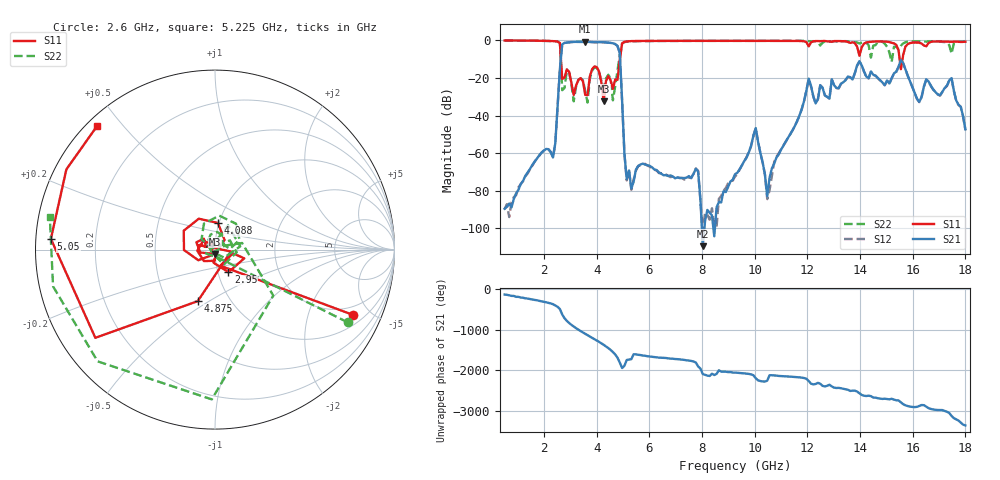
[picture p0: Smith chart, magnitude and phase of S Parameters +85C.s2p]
!Agilent Technologies,N5230A,MY45001468,A.07.50.67
!Agilent N5230A: A.07.50.67
!Date: Thursday, June 27, 2024 16:47:59
!Correction: S11(Full 2 Port(1,2))
!S21(Full 2 Port(1,2))
!S12(Full 2 Port(1,2))
!S22(Full 2 Port(1,2))
!S2P File: Measurements: S11, S21, S12, S22:
# Hz S  dB  R 50
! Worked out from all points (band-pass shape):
!   201 points, 500 MHz to 18 GHz, reference 50 ohm
!   highest |S21| = -0.72 dB at 3.562 GHz (marker M1); lowest = -109.5 dB at 8.025 GHz (marker M2)
!   |S21| within 3 dB of the highest: 2.677 GHz to 4.805 GHz (2.129 GHz wide, 56.9 % of centre)
!   lowest |S11| = -32.5 dB at 4.263 GHz (marker M3), VSWR 1.05, Z = 49.8 - j2.36 ohm
!   |S11| at or under -10 dB: 2.639 GHz to 4.879 GHz (2.239 GHz wide, 59.6 % of centre); 15.5 GHz to 15.61 GHz (107.1 MHz wide, 0.689 % of centre)
!   |S22| runs from -33.1 to 0.0 dB; largest |S21 - S12| = 0.0043
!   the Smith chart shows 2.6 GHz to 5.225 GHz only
!   S11 on the Smith chart (normalised r, x): 2.6 GHz: 1.50, -3.91; 2.95 GHz: 1.12, -0.29; 4.088 GHz: 0.99, +0.30; 4.875 GHz: 0.71, -0.45; 5.05 GHz: 0.04, +0.03; 5.225 GHz: 0.03, +0.43
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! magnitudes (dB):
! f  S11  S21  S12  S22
! 500 MHz  0.0  -89.6  -89.8  0.0
! 2.337 GHz  -0.4  -62.3  -62.2  -0.4
! 2.6 GHz  -1.4  -15.2  -15.2  -1.5
! 2.688 GHz  -20.5  -2.1  -2.1  -26.5
! 2.95 GHz  -16.7  -1.0  -1.0  -17.0
! 3.475 GHz  -21.8  -0.7  -0.8  -21.2
! 3.562 GHz  -29.0  -0.7  -0.7  -26.9
! 4.088 GHz  -16.5  -1.0  -1.0  -16.7
! 4.263 GHz  -32.5  -1.0  -1.0  -25.4
! 4.612 GHz  -25.8  -1.5  -1.5  -31.9
! 4.875 GHz  -10.4  -6.9  -6.9  -7.7
! 5.05 GHz  -0.8  -60.2  -60.3  -0.9
! 5.225 GHz  -0.4  -69.2  -69.0  -0.6
! 6.362 GHz  -0.3  -70.3  -70.7  -0.3
! 8.025 GHz  -0.2  -109.5  -101.9  -0.3
! 9.25 GHz  -0.2  -71.2  -72.5  -0.3
! 10.04 GHz  -0.3  -46.7  -46.7  -0.3
! 10.56 GHz  -0.2  -73.1  -79.7  -0.2
! 12.22 GHz  -0.5  -29.8  -29.9  -0.4
! 15.11 GHz  -0.9  -22.9  -23.1  -6.3
! 17.48 GHz  -0.7  -20.1  -20.2  -7.0
! 18 GHz  -0.7  -47.3  -47.6  -0.5
